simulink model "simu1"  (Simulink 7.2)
settings: Solver=ode45  StartTime=10  StopTime=20  RelTol=1e-3

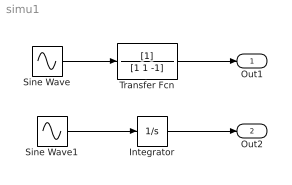
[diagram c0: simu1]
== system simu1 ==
  Integrator : Integrator
  Sine Wave : Sin  SampleTime=0
  Sine Wave1 : Sin  SampleTime=0
  Transfer Fcn : TransferFcn  Denominator=[1 1 -1]
  Out1 : Outport  OutDataType=sfix(16)  OutScaling=2^0
  Out2 : Outport  Port=2  OutDataType=sfix(16)  OutScaling=2^0
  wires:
  Sine Wave/1 -> Transfer Fcn/1
  Transfer Fcn/1 -> Out1/1
  Sine Wave1/1 -> Integrator/1
  Integrator/1 -> Out2/1
